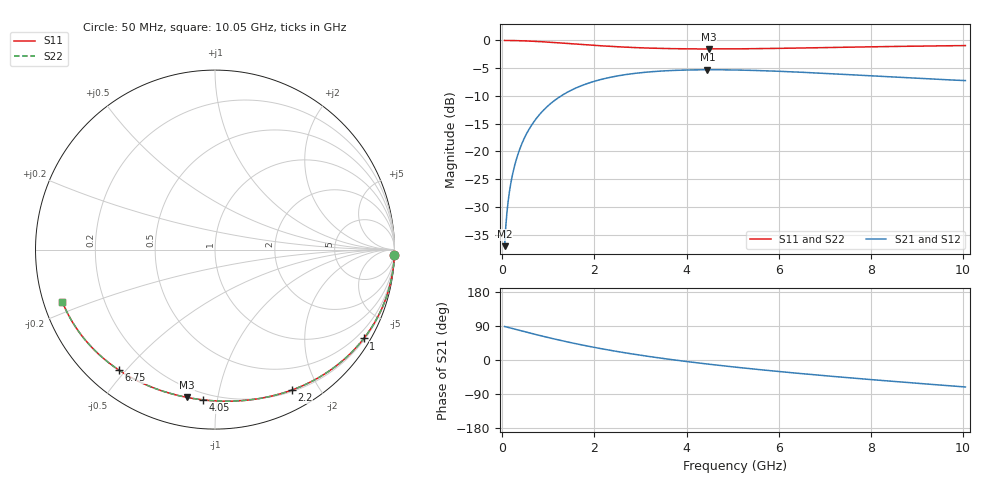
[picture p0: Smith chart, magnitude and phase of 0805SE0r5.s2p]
! AVX Thin Film Operation		Date: August 2001
! Description: Accu-P® Series, Thin Film, SMD, RF Capacitor
! Part Number: 08051J0R5ABT
! 50 MHz  -  10.05 GHz
! Serial Measurements
# mhz S db R 50
!	S11		S21		S12		S22
!	dB	Phase	dB	Phase	dB	Phase	dB	Phase
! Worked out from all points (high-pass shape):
!   401 points, 50 MHz to 10.05 GHz, reference 50 ohm
!   highest |S21| = -5.28 dB at 4.45 GHz (marker M1); lowest = -37.1 dB at 50 MHz (marker M2)
!   |S21| within 3 dB of the highest: 1.679 GHz to end of sweep
!   lowest |S11| = -1.5 dB at 4.475 GHz (marker M3), VSWR 11.35, Z = 7.37 - j40.7 ohm
!   |S11| at or under -10 dB: nowhere
!   |S22| runs from -1.5 to 0.0 dB; largest |S21 - S12| = 6.1e-05
!   S11 on the Smith chart (normalised r, x): 50 MHz: 0, -72; 1 GHz: 0.25, -3.61; 2.2 GHz: 0.22, -1.67; 4.05 GHz: 0.16, -0.91; 6.75 GHz: 0.09, -0.48; 10.05 GHz: 0.05, -0.17
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50  -0.00 -1.6  -37.05 88.4  -37.05 88.4  -0.00 -1.6
75  -0.00 -2.4  -33.53 87.6  -33.53 87.6  -0.00 -2.4
125  -0.01 -4.0  -29.11 86.0  -29.11 86.0  -0.01 -4.0
175  -0.01 -5.6  -26.19 84.4  -26.19 84.4  -0.01 -5.6
250  -0.02 -8.0  -23.12 82.0  -23.12 82.0  -0.02 -8.0
350  -0.04 -11.1  -20.24 78.9  -20.24 78.9  -0.04 -11.1
475  -0.07 -15.0  -17.66 75.0  -17.66 75.0  -0.07 -15.0
625  -0.13 -19.7  -15.39 70.3  -15.39 70.3  -0.13 -19.7
1000  -0.30 -30.8  -11.72 59.2  -11.72 59.2  -0.30 -30.8
1325  -0.49 -39.9  -9.74 50.1  -9.74 50.1  -0.49 -39.9
1725  -0.73 -50.2  -8.12 39.8  -8.12 39.8  -0.73 -50.3
2200  -0.99 -61.3  -6.91 28.7  -6.91 28.7  -0.99 -61.3
2800  -1.26 -73.6  -6.01 16.4  -6.01 16.4  -1.26 -73.6
3400  -1.43 -84.4  -5.54 5.6  -5.54 5.6  -1.43 -84.4
4050  -1.52 -94.7  -5.32 -4.8  -5.32 -4.8  -1.52 -94.8
4450  -1.53 -100.6  -5.28 -10.6  -5.28 -10.6  -1.53 -100.6
4475  -1.53 -100.9  -5.28 -11.0  -5.28 -11.0  -1.53 -101.0
5050  -1.52 -108.7  -5.32 -18.7  -5.32 -18.7  -1.52 -108.7
6725  -1.33 -128.4  -5.82 -38.5  -5.82 -38.5  -1.33 -128.4
6750  -1.32 -128.7  -5.83 -38.8  -5.83 -38.8  -1.32 -128.7
8400  -1.09 -145.5  -6.56 -55.6  -6.56 -55.6  -1.09 -145.5
10050  -0.93 -161.0  -7.23 -71.2  -7.23 -71.2  -0.93 -161.1
